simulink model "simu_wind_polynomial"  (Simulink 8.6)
settings: Solver=ode4  StartTime=0.0  StopTime=runtime  FixedStep=1/fs  RelTol=1e-3
PostLoadFcn:
  | , if any(exist('dsrtsu_mdlpostloadfcn', 'file') == [2, 3, 6]), try dsrtsu_mdlpostloadfcn('Execute', bdroot); catch fprintf('Error in PostLoadFcn (dsrtsu_mdlpostloadfcn) for model "%s":
  |  %s
  | ', bdroot, lasterr); end, end,
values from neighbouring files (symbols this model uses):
  alpha = 0.5    [bowed_string_hyperbolic.m]    (also in polynomial.m = 100)
  an = modal_coeff(:,1)    [hybrid_wind.m]
  delta_cte = 0.1    [polynomial.m]
  Qn = modal_coeff(:,3)    [hybrid_wind.m]
  Ts = 25e-6    (= 2.5e-05)    [hybrid_wind.m]    (also in measurements.m)
  wn = modal_coeff(:,2)    [hybrid_wind.m]
  Zc = rho*c/St    (= 2615281.00417)    [hybrid_wind.m]
  zeta_cte = 0.08    [polynomial.m]
undefined symbols (not defined in the file or in its folder): modal_coeff, vibrato
libraries: simulink x2

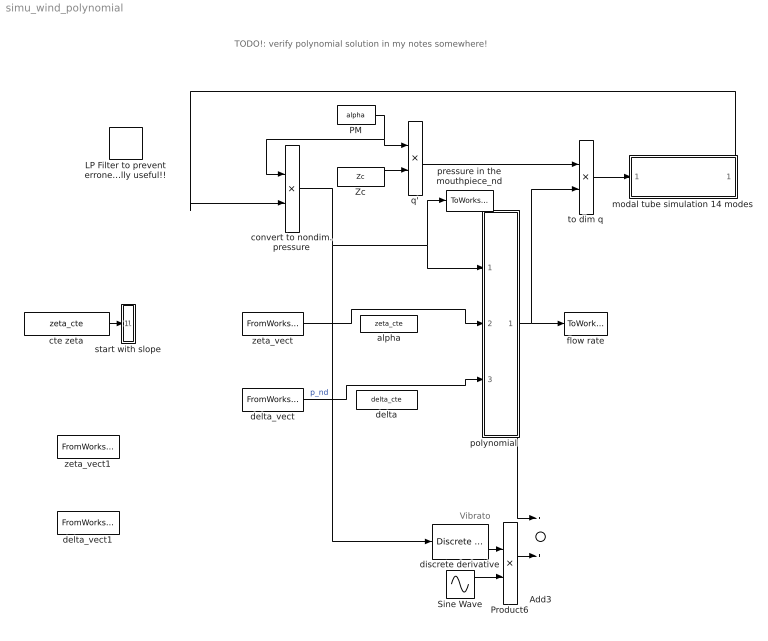
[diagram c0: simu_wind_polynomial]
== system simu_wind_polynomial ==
  note: Vibrato
  note: TODO!: verify polynomial solution in my notes somewhere!
  Add3 : Sum
  LP Filter to prevent erroneous high freq feedback BUT: not really useful!! : DiscreteFilter  Numerator=HdLP.ScaleValues(1)*HdLP.sosMatrix(1:end/2)  Denominator=HdLP.ScaleValues(2)*HdLP.sosMatrix(1+end/2:end)  SampleTime=Ts
  PM : Constant  Value=alpha
  Product6 : Product
  Sine Wave : Sin  Amplitude=vibrato.amp  Bias=-vibrato.amp  Frequency=vibrato.freq*2*pi  SampleTime=0
  Zc : Constant  Value=Zc
  alpha : Constant  Value=zeta_cte
  convert to nondim. pressure : Product  Inputs=/*
  cte zeta : Constant  Value=zeta_cte
  delta : Constant  Value=delta_cte
  delta_vect : FromWorkspace  VariableName=delta_envs_all  SampleTime=Ts  OutputAfterFinalValue=Setting to zero
  delta_vect1 : FromWorkspace  VariableName=delta_vect  SampleTime=Ts  OutputAfterFinalValue=Setting to zero
  discrete derivative : simulink/Discrete/Discrete Derivative  gainval=1.0  ICPrevScaledInput=0.0  InputProcessing=Inherited  OutMin=[]  OutMax=[]  OutDataType=fixdt(1, 16)  OutScaling=2^-10  DoSatur=off
  flow rate : ToWorkspace  VariableName=q_dl  SaveFormat=Structure  SampleTime=-1
  modal tube simulation 14 modes : Subsystem
  polynomial : Subsystem
  pressure in the mouthpiece_nd : ToWorkspace  VariableName=p_dl  SaveFormat=Structure  SampleTime=-1
  q' : Product  Inputs=*/
  start with slope : Subsystem
  to dim q : Product
  zeta_vect : FromWorkspace  VariableName=zeta_envs_all  SampleTime=Ts  OutputAfterFinalValue=Setting to zero
  zeta_vect1 : FromWorkspace  VariableName=zeta_vect  SampleTime=Ts  OutputAfterFinalValue=Setting to zero
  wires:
  Zc/1 -> q'/2
  PM/1 -> convert to nondim. pressure/1, q'/1
  q'/1 -> to dim q/1
  polynomial/1(qdl) -> flow rate/1, to dim q/2, Add3/1
  to dim q/1 -> modal tube simulation 14 modes/1(flowrate_in)
  modal tube simulation 14 modes/1(p_sim_out) -> convert to nondim. pressure/2
  cte zeta/1 -> start with slope/1(cte_in)
  convert to nondim. pressure/1 -> discrete derivative/1, polynomial/1(pdl), pressure in the mouthpiece_nd/1  "p_nd"
  discrete derivative/1 -> Product6/1
  Sine Wave/1 -> Product6/2
  Add3/1 -> ?  "new fdl"
  Product6/1 -> Add3/2
  zeta_vect/1 -> polynomial/2(zeta)
  delta_vect/1 -> polynomial/3(delta)

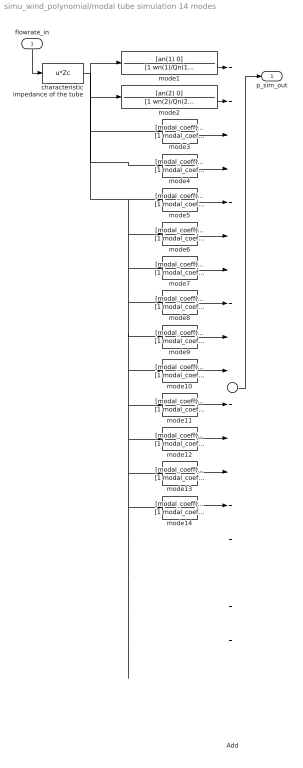
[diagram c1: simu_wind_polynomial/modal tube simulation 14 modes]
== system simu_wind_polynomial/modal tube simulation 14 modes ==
  flowrate_in : Inport
  Add : Sum  Inputs=++++++++++++++++++++
  characteristic impedance of the tube : Fcn  Expr=u*Zc
  mode1 : TransferFcn  Numerator=[an(1) 0]  Denominator=[1 wn(1)/Qn(1) wn(1)^2]
  mode10 : TransferFcn  Numerator=[modal_coeff(10, 1) 0]  Denominator=[1 modal_coeff(10,2)/modal_coeff(10,3) modal_coeff(10,2)^2]
  mode11 : TransferFcn  Numerator=[modal_coeff(11, 1) 0]  Denominator=[1 modal_coeff(11,2)/modal_coeff(11,3) modal_coeff(11,2)^2]
  mode12 : TransferFcn  Numerator=[modal_coeff(12, 1) 0]  Denominator=[1 modal_coeff(12,2)/modal_coeff(12,3) modal_coeff(12,2)^2]
  mode13 : TransferFcn  Numerator=[modal_coeff(13, 1) 0]  Denominator=[1 modal_coeff(13,2)/modal_coeff(13,3) modal_coeff(13,2)^2]
  mode14 : TransferFcn  Numerator=[modal_coeff(14, 1) 0]  Denominator=[1 modal_coeff(14,2)/modal_coeff(14,3) modal_coeff(14,2)^2]
  mode2 : TransferFcn  Numerator=[an(2) 0]  Denominator=[1 wn(2)/Qn(2) wn(2)^2]
  mode3 : TransferFcn  Numerator=[modal_coeff(3, 1) 0]  Denominator=[1 modal_coeff(3,2)/modal_coeff(3,3) modal_coeff(3,2)^2]
  mode4 : TransferFcn  Numerator=[modal_coeff(4, 1) 0]  Denominator=[1 modal_coeff(4,2)/modal_coeff(4,3) modal_coeff(4,2)^2]
  mode5 : TransferFcn  Numerator=[modal_coeff(5, 1) 0]  Denominator=[1 modal_coeff(5,2)/modal_coeff(5,3) modal_coeff(5,2)^2]
  mode6 : TransferFcn  Numerator=[modal_coeff(6, 1) 0]  Denominator=[1 modal_coeff(6,2)/modal_coeff(6,3) modal_coeff(6,2)^2]
  mode7 : TransferFcn  Numerator=[modal_coeff(7, 1) 0]  Denominator=[1 modal_coeff(7,2)/modal_coeff(7,3) modal_coeff(7,2)^2]
  mode8 : TransferFcn  Numerator=[modal_coeff(8, 1) 0]  Denominator=[1 modal_coeff(8,2)/modal_coeff(8,3) modal_coeff(8,2)^2]
  mode9 : TransferFcn  Numerator=[modal_coeff(9, 1) 0]  Denominator=[1 modal_coeff(9,2)/modal_coeff(9,3) modal_coeff(9,2)^2]
  p_sim_out : Outport
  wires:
  flowrate_in/1 -> characteristic impedance of the tube/1
  characteristic impedance of the tube/1 -> mode4/1, mode3/1, mode2/1, mode1/1, mode5/1, mode6/1, mode7/1, mode8/1, mode9/1, mode10/1, mode11/1, mode12/1, mode13/1, mode14/1
  mode1/1 -> Add/1
  Add/1 -> p_sim_out/1
  mode2/1 -> Add/2
  mode3/1 -> Add/3
  mode4/1 -> Add/4
  mode5/1 -> Add/5
  mode6/1 -> Add/6
  mode7/1 -> Add/7
  mode8/1 -> Add/8
  mode9/1 -> Add/9
  mode10/1 -> Add/10
  mode11/1 -> Add/11
  mode12/1 -> Add/12
  mode13/1 -> Add/13
  ? -> Add/15
  mode14/1 -> Add/14

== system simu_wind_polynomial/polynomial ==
  pdl : Inport
  zeta : Inport  Port=2
  delta : Inport  Port=3
  Add3 : Sum  Inputs=-+
  Unit Delay : UnitDelay  SampleTime=-1
  calc. real root of 3rd order eq ->old! : Subsystem
  implicit to explicit + calc real root of 3rd order eq. : S-Function  InitFcn=try, set_param(gcb,'FunctionName','polynomial_excitation'), end  FunctionName=polynomial_excitation  SFunctionModules=polynomial_excitation_wrapper  WizardData=DataTag0  SFunctionDeploymentMode=off  EnableBusSupport=off
  qdl : Outport
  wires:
  zeta/1 -> implicit to explicit + calc real root of 3rd order eq./2
  delta/1 -> implicit to explicit + calc real root of 3rd order eq./3
  implicit to explicit + calc real root of 3rd order eq./1 -> Unit Delay/1, qdl/1
  Add3/1 -> implicit to explicit + calc real root of 3rd order eq./1  "pretneding to be phdl but is actually phdl\u001dn-1"
  pdl/1 -> Add3/2
  Unit Delay/1 -> Add3/1  "approximative q[n]"

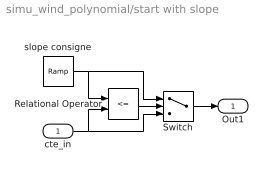
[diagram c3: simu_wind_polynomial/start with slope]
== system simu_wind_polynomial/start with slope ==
  cte_in : Inport
  Relational Operator : RelationalOperator  Operator=<=  OutDataTypeStr=boolean
  Switch : Switch  Criteria=u2 > Threshold
  slope consigne : simulink/Sources/Ramp  slope=zeta_cte*100  start=0  X0=0
  Out1 : Outport
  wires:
  slope consigne/1 -> Relational Operator/1, Switch/1
  cte_in/1 -> Relational Operator/2, Switch/3
  Relational Operator/1 -> Switch/2
  Switch/1 -> Out1/1

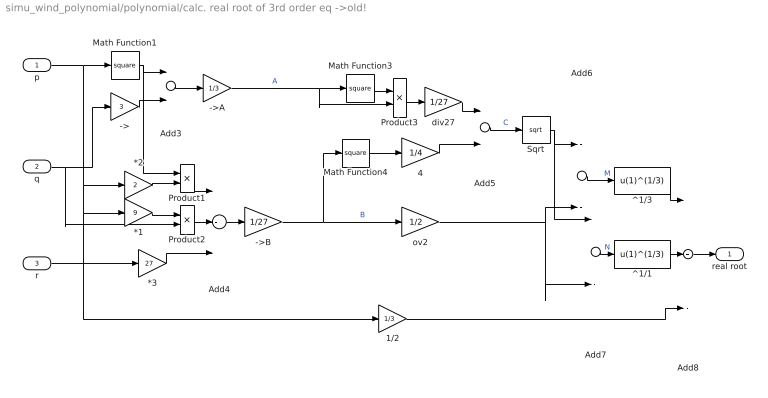
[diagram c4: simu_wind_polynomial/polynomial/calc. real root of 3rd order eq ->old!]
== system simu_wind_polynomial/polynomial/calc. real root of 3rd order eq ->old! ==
  p : Inport
  q : Inport  Port=2
  r : Inport  Port=3
  *1 : Gain  Gain=9
  *2 : Gain  Gain=2
  *3 : Gain  Gain=27
  -> : Gain  Gain=3
  ->A : Gain  Gain=1/3
  ->B : Gain  Gain=1/27
  1/2 : Gain  Gain=1/3
  4 : Gain  Gain=1/4
  Add3 : Sum  Inputs=-+
  Add4 : Sum  Inputs=+-+
  Add5 : Sum
  Add6 : Sum  Inputs=+-
  Add7 : Sum  Inputs=--
  Add8 : Sum  Inputs=++-
  Math Function1 : Math  Operator=square
  Math Function3 : Math  Operator=square
  Math Function4 : Math  Operator=square
  Product1 : Product
  Product2 : Product
  Product3 : Product
  Sqrt : Sqrt
  ^1/1 : Fcn  Expr=u(1)^(1/3)
  ^1/3 : Fcn  Expr=u(1)^(1/3)
  div27 : Gain  Gain=1/27
  ov2 : Gain  Gain=1/2
  real root : Outport
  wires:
  p/1 -> 1/2/1, *1/1, *2/1, Math Function1/1
  q/1 -> Product2/2, ->/1
  Math Function1/1 -> Add3/1, Product1/1
  ->/1 -> Add3/2
  Add3/1 -> ->A/1
  ->A/1 -> Math Function3/1, Product3/2  "A"
  Product1/1 -> Add4/1
  Add4/1 -> ->B/1
  ->B/1 -> Math Function4/1, ov2/1  "B"
  *2/1 -> Product1/2
  Product2/1 -> Add4/2
  *1/1 -> Product2/1
  *3/1 -> Add4/3
  Math Function3/1 -> Product3/1
  Product3/1 -> div27/1
  div27/1 -> Add5/1
  Math Function4/1 -> 4/1
  4/1 -> Add5/2
  Add5/1 -> Sqrt/1  "C"
  Sqrt/1 -> Add6/1, Add7/1
  ov2/1 -> Add6/2, Add7/2
  1/2/1 -> Add8/3
  Add6/1 -> ^1/3/1  "M"
  ^1/3/1 -> Add8/1
  Add7/1 -> ^1/1/1  "N"
  ^1/1/1 -> Add8/2
  Add8/1 -> real root/1
  r/1 -> *3/1
